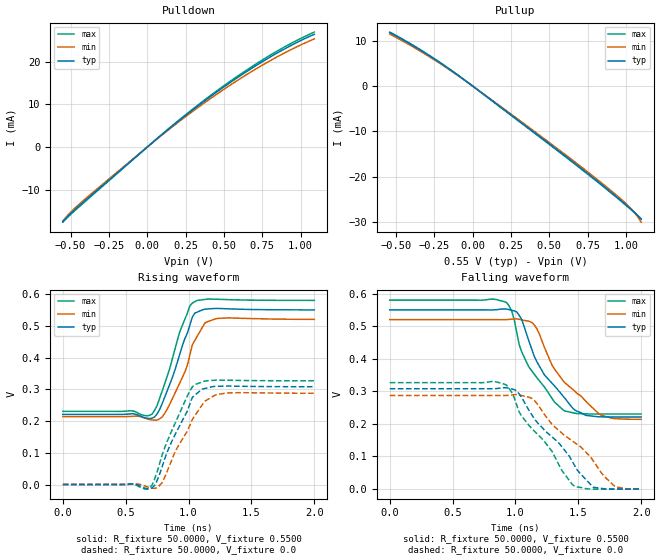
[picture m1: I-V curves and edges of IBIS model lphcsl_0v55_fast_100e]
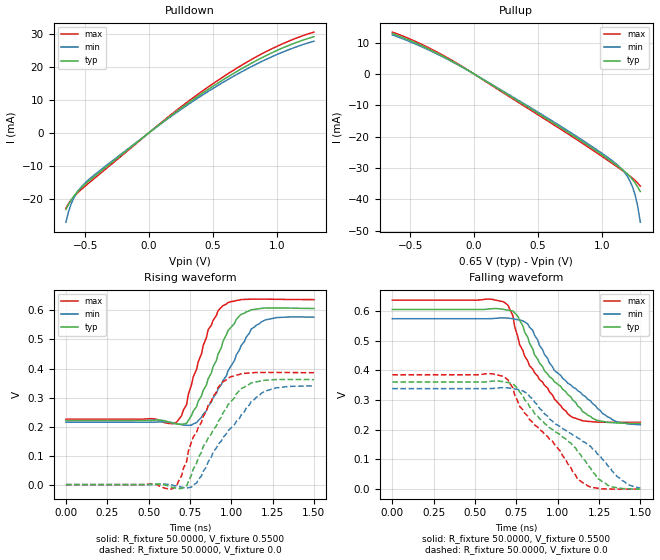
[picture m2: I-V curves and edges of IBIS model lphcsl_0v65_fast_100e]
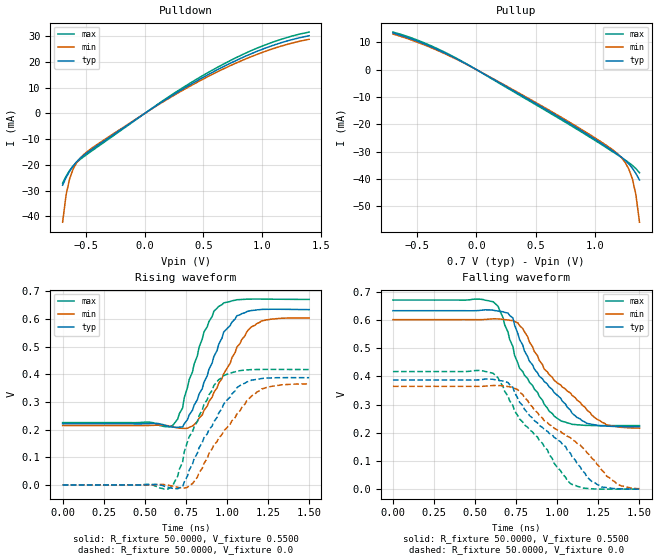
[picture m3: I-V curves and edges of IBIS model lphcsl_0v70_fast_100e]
| Integrated Devices Technolgy, Inc
[IBIS Ver]   4.1
[File name]   9fgl08p1.ibs
[File Rev]   1.0
|Rev history   1.0   original ibis data
[Date]   17 March, 2016
[Disclaimer] Integrated Device Technology, Inc. ("IDT") hereby grants the
   user of this ibis model a non-exclusive, nontransferable
   license to use this ibis model under the following terms. the
   user is granted this license only to use the ibis model and is
   not granted rights to sell, copy (except as needed to run the
   ibis model), rent, lease or sub-license the ibis model in
   whole or in part, or in modified form to anyone. the user may
   modify the ibis model to suit its specific applications, but
   rights to derivative works and such modifications shall belong
   to idt. this ibis model is provided on an as is" basis and idt
   makes absolutely no warranty with respect to the information
   contained herein. idt disclaims and customer waives all
   warranties, express and implied, including warranties of
   merchantability and fitness for a particular purpose. the
   entire risk as to quality and performance is with the user
   accordingly, in no event shall idt be liable for any direct or
   indirect damages, whether in contract or tort, including any
   lost profits or other incidental, consequential, exemplary, or
   punitive damages arising out of the use or application of the
   ibis model. further, idt reserves the right to make changes
   without notice to any product herein to improve reliability,
   function, or design. idt does not convey any license under
   patent rights or any other intellectual property rights,
   including those of third parties. idt is not obligated to
   provide maintenance or support for the licensed ibis model.
[Copyright]   Copyright 2012, Integrated Devices Technolgy, Inc. all rights
   reserved
[Component]   9fgl08p1
[Manufacturer] Integrated Device Technology, Inc.
[Package]
R_pkg   72.4655m   58.886m   86.045m
L_pkg   1.47175nH   1.11650nH   1.77850nH
C_pkg   0.07747pF   0.07444pF   0.08050pF
[Pin] signal_name  model_name
1   vSS_EN_tri   GND
2   GNDXTAL   GND
3   XIN/CLKIN_25   X1
4   X2   X2
5   VDDXTAL3.3   POWER
6   VDDREF3.3   POWER
7   vSADR/REF3.3   REF
8   GNDREF   GND
9   GNDDIG   GND
10   SCLK_3.3   SCIN
11   SDATA_3.3   SCIN
12   VDDDIG3.3   POWER
13   VDDIO   POWER
14   vOE0#   IN
15   DIF0   LP_HCSL
16   DIF0#   LP_HCSL
17   vOE1#   IN
18   DIF1   LP_HCSL
19   DIF1#   LP_HCSL
20   VDD3.3   POWER
21   VDDIO   POWER
22   GND   GND
23   DIF2   LP_HCSL
24   DIF2#   LP_HCSL
25   vOE2#   IN
26   DIF3   LP_HCSL
27   DIF3#   LP_HCSL
28   vOE3#   IN
29   GNDA   GND
30   VDDA3.3   POWER
31   VDDIO   POWER
32   DIF4   LP_HCSL
33   DIF4#   LP_HCSL
34   vOE4#   IN
35   DIF5   LP_HCSL
36   DIF5#   LP_HCSL
37   vOE5#   IN
38   VDD3.3   POWER
39   VDDIO   POWER
40   GND   GND
41   DIF6   LP_HCSL
42   DIF6#   LP_HCSL
43   vOE6#   IN
44   DIF7   LP_HCSL
45   DIF7#   LP_HCSL
46   vOE7#   IN
47   VDDIO   POWER
48   ^CKPWRGD_PD#   PD
49   ePAD   GND
[Diff Pin]  inv_pin  vdiff tdelay_typ tdelay_min  tdelay_max
15   16   NA   0   0   0
18   19   NA   0   0   0
23   24   NA   0   0   0
26   27   NA   0   0   0
32   33   NA   0   0   0
35   36   NA   0   0   0
41   42   NA   0   0   0
44   45   NA   0   0   0
[Model Selector] LP_HCSL
lphcsl_0v55_fast_33e amplitude 0.55V, slew rate fast, 33 ohm diff impedance
lphcsl_0v55_slow_33e amplitude 0.55V, slew rate slow, 33 ohm diff impedance
lphcsl_0v65_fast_33e amplitude 0.65V, slew rate fast, 33 ohm diff impedance
lphcsl_0v65_slow_33e amplitude 0.65V, slew rate slow, 33 ohm diff impedance
lphcsl_0v70_fast_33e amplitude 0.70V, slew rate fast, 33 ohm diff impedance
lphcsl_0v70_slow_33e amplitude 0.70V, slew rate slow, 33 ohm diff impedance
lphcsl_0v80_fast_33e amplitude 0.80V, slew rate fast, 33 ohm diff impedance
lphcsl_0v80_slow_33e amplitude 0.80V, slew rate slow, 33 ohm diff impedance
lphcsl_0v55_fast_85e amplitude 0.55V, slew rate fast, 85 ohm diff impedance
lphcsl_0v55_slow_85e amplitude 0.55V, slew rate slow, 85 ohm diff impedance
lphcsl_0v65_fast_85e amplitude 0.65V, slew rate fast, 85 ohm diff impedance
lphcsl_0v65_slow_85e amplitude 0.65V, slew rate slow, 85 ohm diff impedance
lphcsl_0v70_fast_85e amplitude 0.70V, slew rate fast, 85 ohm diff impedance
lphcsl_0v70_slow_85e amplitude 0.70V, slew rate slow, 85 ohm diff impedance
lphcsl_0v80_fast_85e amplitude 0.80V, slew rate fast, 85 ohm diff impedance
lphcsl_0v80_slow_85e amplitude 0.80V, slew rate slow, 85 ohm diff impedance
lphcsl_0v55_fast_100e amplitude 0.55V, slew rate fast, 100 ohm diff impedance
lphcsl_0v55_slow_100e amplitude 0.55V, slew rate slow, 100 ohm diff impedance
lphcsl_0v65_fast_100e amplitude 0.65V, slew rate fast, 100 ohm diff impedance
lphcsl_0v65_slow_100e amplitude 0.65V, slew rate slow, 100 ohm diff impedance
lphcsl_0v70_fast_100e amplitude 0.70V, slew rate fast, 100 ohm diff impedance
lphcsl_0v70_slow_100e amplitude 0.70V, slew rate slow, 100 ohm diff impedance
lphcsl_0v80_fast_100e amplitude 0.80V, slew rate fast, 100 ohm diff impedance
lphcsl_0v80_slow_100e amplitude 0.80V, slew rate slow, 100 ohm diff impedance
| Models and submodels in the file (30): REF (Output), lphcsl_0v55_fast_100e (Output), lphcsl_0v55_slow_100e (Output), lphcsl_0v65_fast_100e (Output), lphcsl_0v65_slow_100e (Output), lphcsl_0v70_fast_100e (Output), lphcsl_0v70_slow_100e (Output), lphcsl_0v80_fast_100e (Output), lphcsl_0v80_slow_100e (Output), lphcsl_0v55_fast_85e (Output), lphcsl_0v55_slow_85e (Output), lphcsl_0v65_fast_85e (Output), lphcsl_0v65_slow_85e (Output), lphcsl_0v70_fast_85e (Output), lphcsl_0v70_slow_85e (Output), lphcsl_0v80_fast_85e (Output), lphcsl_0v80_slow_85e (Output), lphcsl_0v55_fast_33e (Output), lphcsl_0v55_slow_33e (Output), lphcsl_0v65_fast_33e (Output), lphcsl_0v65_slow_33e (Output), lphcsl_0v70_fast_33e (Output), lphcsl_0v70_slow_33e (Output), lphcsl_0v80_fast_33e (Output), lphcsl_0v80_slow_33e (Output), SCIN (Input), IN (Input), PD (Input), X1 (Input), X2 (Output)
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[Model]   lphcsl_0v55_fast_100e
Model_type Output
Polarity   Non-Inverting
Enable   Active-High
Vmeas =  0.4000V
Cref =   2.0000pF
Rref =   0.0
Vref =   0.4000V
C_comp   1.1000pF   1.0000pF   1.2000pF
[Temperature Range]   25.0000   85.0000   -40.0
[Voltage Range]   0.5500V   0.5200V   0.5800V
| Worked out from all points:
|   slope of the pulldown table from 0 to 0.083 V, typ, clamps not added: 32.7 ohm
|   slope of the pullup table from 0 to 0.083 V, typ, clamps not added: 39.3 ohm
|   rising waveform, R_fixture 50.0000, V_fixture 0.5500: 20-80 % time 174ps typ, 180ps min, 165ps max; typ from 0.221 V to 0.55 V
|   rising waveform, R_fixture 50.0000, V_fixture 0.0: 20-80 % time 210ps typ, 226ps min, 201ps max; typ from 0 V to 0.308 V
|   falling waveform, R_fixture 50.0000, V_fixture 0.5500: 20-80 % time 295ps typ, 339ps min, 258ps max; typ from 0.55 V to 0.221 V
|   falling waveform, R_fixture 50.0000, V_fixture 0.0: 20-80 % time 385ps typ, 441ps min, 351ps max; typ from 0.308 V to 0 V
[Pulldown]
|Voltage   I(typ)   I(min)   I(max)
-550mV    -17.42mA   -17.31mA   -17.56mA
-510mV    -15.92mA   -15.61mA   -16.12mA
-470mV    -14.59mA   -14.21mA   -14.8mA
-310mV    -9.584mA   -9.264mA   -9.753mA
90mV      2.747mA    2.637mA    2.806mA
350mV     10.16mA    9.756mA    10.37mA
570mV     15.8mA     15.17mA    16.12mA
750mV     19.95mA    19.15mA    20.36mA
910mV     23.24mA    22.29mA    23.72mA
1.09V     26.39mA    25.32mA    26.91mA
[Pullup]
|Voltage   I(typ)   I(min)   I(max)
-540mV    11.78mA    11.45mA    11.88mA
-360mV    8.313mA    8.057mA    8.417mA
-160mV    3.912mA    3.778mA    3.974mA
0V        -107.6pA   -683pA     -85.53pA
480mV     -12.23mA   -11.94mA   -12.36mA
760mV     -19.55mA   -19.19mA   -19.69mA
960mV     -25.05mA   -24.7mA    -25.17mA
1.04V     -27.39mA   -27.28mA   -27.47mA
1.08V     -28.69mA   -28.98mA   -28.66mA
1.1V      -29.42mA   -30.05mA   -29.29mA
[Ramp]
| variable   typ   min   max
dV/dt_r  0.1848/0.2165n   0.1724/0.2461n   0.1960/0.2011n
dV/dt_f  0.1973/0.2848n   0.1835/0.3291n   0.2098/0.2758n
R_load = 50.0000
[Rising Waveform]
R_fixture= 50.0000
V_fixture= 0.5500
V_fixture_min= 0.5200
V_fixture_max= 0.5800
|time   V(typ)   V(min)   V(max)
0s        221mV      213.9mV    230.4mV
710ps     208.9mV    203.3mV    222mV
770ps     236.5mV    207.1mV    271.8mV
830ps     295.1mV    237.4mV    341.4mV
930ps     410.6mV    320mV      481.3mV
1.01ns    502mV      407.6mV    562.8mV
1.07ns    543.3mV    467.9mV    580.1mV
1.13ns    552.4mV    509.1mV    583mV
1.23ns    554.6mV    523.3mV    583.5mV
2ns       550.1mV    520.2mV    580mV
[Rising Waveform]
R_fixture= 50.0000
V_fixture= 0.0
V_fixture_min= 0.0
V_fixture_max= 0.0
|time   V(typ)   V(min)   V(max)
0s        0V         0V         0V
690ps     -13.76mV   -9.908mV   -11mV
730ps     -2.555mV   -12mV      17.28mV
790ps     56.31mV    6.206mV    93.42mV
890ps     155mV      100.6mV    190.4mV
990ps     231mV      167.8mV    278.9mV
1.05ns    281.3mV    216.8mV    314.6mV
1.13ns    302.4mV    262.5mV    326.1mV
1.23ns    309.3mV    283.7mV    328.7mV
2ns       308mV      287.4mV    326.7mV
[Falling Waveform]
R_fixture= 50.0000
V_fixture= 0.5500
V_fixture_min= 0.5200
V_fixture_max= 0.5800
|time   V(typ)   V(min)   V(max)
0s        550mV      520mV      580mV
930ps     552.4mV    520.1mV    572.5mV
970ps     548.8mV    521.6mV    546.6mV
1.03ns    533mV      521mV      442.9mV
1.11ns    451.2mV    514.7mV    373mV
1.23ns    350.6mV    435.4mV    313.4mV
1.31ns    317mV      368.9mV    267.2mV
1.47ns    243.2mV    301.1mV    233mV
1.68ns    221.7mV    226.8mV    230.4mV
2ns       221.1mV    214.1mV    230.4mV
[Falling Waveform]
R_fixture= 50.0000
V_fixture= 0.0
V_fixture_min= 0.0
V_fixture_max= 0.0
|time   V(typ)   V(min)   V(max)
0s        307.9mV    287.3mV    326.7mV
890ps     310.7mV    287.1mV    324.6mV
950ps     309.3mV    287.8mV    308.9mV
1.01ns    301.5mV    290mV      257.9mV
1.11ns    240.4mV    281.8mV    194.3mV
1.29ns    160.4mV    199.1mV    116.1mV
1.47ns    72.59mV    142.7mV    8.438mV
1.62ns    5.493mV    86.02mV    77.42uV
1.78ns    -65.96uV   11.35mV    -85.75uV
2ns       -77.45uV   -198.5uV   -34.61uV
[Model]   lphcsl_0v65_fast_100e
Model_type Output
Polarity   Non-Inverting
Enable   Active-High
Vmeas =  0.4000V
Cref =   2.0000pF
Rref =   0.0
Vref =   0.4000V
C_comp   1.1000pF   1.0000pF   1.2000pF
[Temperature Range]   25.0000   85.0000   -40.0000
[Voltage Range]   0.6500V   0.6200V   0.6800V
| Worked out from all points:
|   slope of the pulldown table from 0 to 0.098 V, typ, clamps not added: 32.8 ohm
|   slope of the pullup table from 0 to 0.098 V, typ, clamps not added: 40 ohm
|   rising waveform, R_fixture 50.0000, V_fixture 0.5500: 20-80 % time 168ps typ, 206ps min, 144ps max; typ from 0.221 V to 0.607 V
|   rising waveform, R_fixture 50.0000, V_fixture 0.0: 20-80 % time 214ps typ, 251ps min, 168ps max; typ from 0 V to 0.362 V
|   falling waveform, R_fixture 50.0000, V_fixture 0.5500: 20-80 % time 294ps typ, 332ps min, 239ps max; typ from 0.606 V to 0.222 V
|   falling waveform, R_fixture 50.0000, V_fixture 0.0: 20-80 % time 376ps typ, 429ps min, 326ps max; typ from 0.361 V to 0 V
[Pulldown]
|Voltage   I(typ)   I(min)   I(max)
-650mV    -23.23mA   -27.08mA   -22.85mA
-630mV    -21.73mA   -23.92mA   -21.53mA
-610mV    -20.42mA   -21.63mA   -20.41mA
-590mV    -19.28mA   -19.88mA   -19.45mA
-550mV    -17.42mA   -17.37mA   -17.87mA
-510mV    -15.92mA   -15.58mA   -16.5mA
-350mV    -10.82mA   -10.4mA    -11.34mA
130mV     3.938mA    3.75mA     4.173mA
450mV     12.8mA     12.19mA    13.51mA
770mV     20.38mA    19.39mA    21.48mA
1.03V     25.42mA    24.16mA    26.67mA
1.29V     29.08mA    27.71mA    30.47mA
[Pullup]
|Voltage   I(typ)   I(min)   I(max)
-640mV    12.9mA     12.48mA    13.37mA
-340mV    7.668mA    7.369mA    8.057mA
-40mV     988uA      943.5uA    1.052mA
700mV     -17.66mA   -17.23mA   -18.19mA
1.08V     -28.05mA   -27.62mA   -28.49mA
1.16V     -30.49mA   -30.54mA   -30.78mA
1.2V      -31.91mA   -32.71mA   -31.96mA
1.22V     -32.74mA   -34.19mA   -32.58mA
1.24V     -33.69mA   -36.08mA   -33.24mA
1.26V     -34.78mA   -38.62mA   -33.96mA
1.28V     -36.03mA   -42.17mA   -34.78mA
1.3V      -37.46mA   -47.25mA   -35.74mA
[Ramp]
| variable   typ   min   max
dV/dt_r  0.2171/0.2129n   0.2039/0.2456n   0.2314/0.1862n
dV/dt_f  0.2322/0.2706n   0.2162/0.3099n   0.2487/0.2338n
R_load = 50.0000
[Rising Waveform]
R_fixture= 50.0000
V_fixture= 0.5500
V_fixture_min= 0.5200
V_fixture_max= 0.5800
|time   V(typ)   V(min)   V(max)
0s        221mV      214.9mV    225.3mV
650ps     210.5mV    212.1mV    210.1mV
730ps     211.4mV    204.5mV    276.1mV
790ps     268.6mV    213.4mV    396.8mV
860ps     364.5mV    269.7mV    533.4mV
950ps     494mV      359.2mV    616.5mV
1.05ns    581.6mV    464.5mV    635.9mV
1.15ns    604.7mV    548.6mV    639.1mV
1.27ns    608.6mV    575.2mV    638.3mV
1.5ns     606.8mV    576.9mV    637.3mV
[Rising Waveform]
R_fixture= 50.0000
V_fixture= 0.0
V_fixture_min= 0.0
V_fixture_max= 0.0
|time   V(typ)   V(min)   V(max)
0s        0V         0V         0V
640ps     -8.434mV   -704uV     -15.02mV
700ps     -13.35mV   -8.846mV   31.11mV
730ps     -5.209mV   -11.48mV   79.09mV
760ps     34.44mV    -8.318mV   147.9mV
790ps     73.04mV    5.508mV    180.3mV
950ps     247.4mV    162.6mV    354.6mV
1.06ns    330.8mV    239.9mV    381.8mV
1.2ns     359.3mV    320.7mV    386.4mV
1.5ns     361.8mV    339.9mV    385.6mV
[Falling Waveform]
R_fixture= 50.0000
V_fixture= 0.5500
V_fixture_min= 0.5200
V_fixture_max= 0.5800
|time   V(typ)   V(min)   V(max)
0s        605.5mV    574.4mV    637mV
610ps     608.4mV    574.9mV    639.2mV
730ps     600.1mV    574.5mV    584.1mV
770ps     569.5mV    570.1mV    487.1mV
830ps     491.6mV    545.6mV    416.2mV
920ps     399.1mV    454.6mV    350.4mV
1.06ns    319.5mV    357.6mV    254.3mV
1.23ns    233.7mV    280.6mV    226.2mV
1.36ns    223mV      226.1mV    225.3mV
1.5ns     221.5mV    216.9mV    225.3mV
[Falling Waveform]
R_fixture= 50.0000
V_fixture= 0.0
V_fixture_min= 0.0
V_fixture_max= 0.0
|time   V(typ)   V(min)   V(max)
0s        361mV      338.8mV    385.4mV
610ps     364mV      339.3mV    388.2mV
680ps     360.8mV    341.6mV    377mV
730ps     355.5mV    339.4mV    341.2mV
770ps     327.7mV    334.4mV    279.2mV
970ps     200.9mV    228.4mV    160.8mV
1.12ns    126.5mV    172.8mV    33.06mV
1.3ns     13.89mV    80.88mV    422.7uV
1.42ns    1.232mV    16.25mV    -179.8uV
1.5ns     169.3uV    3.586mV    -100uV
[Model]   lphcsl_0v70_fast_100e
Model_type Output
Polarity   Non-Inverting
Enable   Active-High
Vmeas =  0.4000V
Cref =   2.0000pF
Rref =   0.0
Vref =   0.4000V
C_comp   1.1000pF   1.0000pF   1.2000pF
[Temperature Range]   25.0000   85.0000   -40.0000
[Voltage Range]   0.7000V   0.6700V   0.7400V
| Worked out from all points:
|   slope of the pulldown table from 0 to 0.105 V, typ, clamps not added: 32.9 ohm
|   slope of the pullup table from 0 to 0.105 V, typ, clamps not added: 40.5 ohm
|   rising waveform, R_fixture 50.0000, V_fixture 0.5500: 20-80 % time 164ps typ, 205ps min, 146ps max; typ from 0.221 V to 0.634 V
|   rising waveform, R_fixture 50.0000, V_fixture 0.0: 20-80 % time 214ps typ, 252ps min, 170ps max; typ from 0 V to 0.388 V
|   falling waveform, R_fixture 50.0000, V_fixture 0.5500: 20-80 % time 286ps typ, 333ps min, 230ps max; typ from 0.633 V to 0.221 V
|   falling waveform, R_fixture 50.0000, V_fixture 0.0: 20-80 % time 372ps typ, 416ps min, 296ps max; typ from 0.387 V to 0 V
[Pulldown]
|Voltage   I(typ)   I(min)   I(max)
-700mV    -27.91mA   -42.29mA   -27.13mA
-670mV    -24.93mA   -31.58mA   -24.4mA
-640mV    -22.46mA   -25.38mA   -22.16mA
-610mV    -20.43mA   -21.63mA   -20.41mA
-550mV    -17.42mA   -17.37mA   -17.87mA
-460mV    -14.27mA   -13.81mA   -14.87mA
170mV     5.111mA    4.867mA    5.413mA
620mV     17mA       16.18mA    17.92mA
830mV     21.65mA    20.59mA    22.8mA
1.01V     25.07mA    23.84mA    26.32mA
1.22V     28.24mA    26.89mA    29.6mA
1.4V      30.17mA    28.8mA     31.59mA
[Pullup]
|Voltage   I(typ)   I(min)   I(max)
-700mV    13.37mA    12.97mA    13.69mA
-400mV    8.685mA    8.356mA    9.067mA
-40mV     976.3uA    932.1uA    1.037mA
710mV     -17.77mA   -17.34mA   -18.25mA
1.01V     -25.83mA   -25.34mA   -26.25mA
1.16V     -30.15mA   -29.81mA   -30.44mA
1.22V     -32.05mA   -32.24mA   -32.17mA
1.25V     -33.15mA   -33.95mA   -33.06mA
1.28V     -34.44mA   -36.32mA   -33.98mA
1.31V     -36.02mA   -39.87mA   -35mA
1.34V     -37.97mA   -45.72mA   -36.19mA
1.37V     -40.34mA   -55.75mA   -37.7mA
[Ramp]
| variable   typ   min   max
dV/dt_r  0.2327/0.2120n   0.2192/0.2438n   0.2503/0.1864n
dV/dt_f  0.2497/0.2565n   0.2337/0.2967n   0.2701/0.2197n
R_load = 50.0000
[Rising Waveform]
R_fixture= 50.0000
V_fixture= 0.5500
V_fixture_min= 0.5200
V_fixture_max= 0.5800
|time   V(typ)   V(min)   V(max)
0s        221mV      214.9mV    225.3mV
650ps     210.9mV    212.4mV    210.2mV
730ps     209.9mV    204.6mV    278mV
800ps     288.3mV    217.9mV    436.5mV
860ps     371.3mV    269.2mV    553.3mV
950ps     508.9mV    368mV      645.7mV
1.06ns    611.8mV    498mV      669.8mV
1.15ns    630.9mV    572mV      672.2mV
1.24ns    635.1mV    597mV      672mV
1.5ns     634mV      603.5mV    671mV
[Rising Waveform]
R_fixture= 50.0000
V_fixture= 0.0
V_fixture_min= 0.0
V_fixture_max= 0.0
|time   V(typ)   V(min)   V(max)
0s        0V         0V         0V
640ps     -8.091mV   -315uV     -15.03mV
670ps     -12.45mV   -4.428mV   -2.669mV
730ps     -7.069mV   -11.24mV   81.56mV
770ps     53.48mV    -3.061mV   174.1mV
860ps     170.1mV    77.73mV    291.3mV
980ps     292.4mV    195mV      395.2mV
1.09ns    363.9mV    280.3mV    414.1mV
1.21ns    384.8mV    347.2mV    417.7mV
1.5ns     387.8mV    365.3mV    417.2mV
[Falling Waveform]
R_fixture= 50.0000
V_fixture= 0.5500
V_fixture_min= 0.5200
V_fixture_max= 0.5800
|time   V(typ)   V(min)   V(max)
0s        632.9mV    601.2mV    670.7mV
610ps     634.7mV    604mV      664.5mV
640ps     631.8mV    603.8mV    648.2mV
730ps     606.8mV    597.8mV    505.4mV
770ps     531.2mV    580.1mV    429.2mV
830ps     454.4mV    522.4mV    379.2mV
950ps     363mV      406.2mV    276.6mV
1.12ns    254.1mV    315.7mV    228.3mV
1.3ns     223.5mV    227.5mV    225.4mV
1.5ns     221.4mV    216.3mV    225.3mV
[Falling Waveform]
R_fixture= 50.0000
V_fixture= 0.0
V_fixture_min= 0.0
V_fixture_max= 0.0
|time   V(typ)   V(min)   V(max)
0s        387.1mV    364.6mV    417.1mV
610ps     389.4mV    367.5mV    410.7mV
730ps     361.1mV    361.3mV    296.8mV
830ps     261mV      302.3mV    210.9mV
920ps     212mV      242.7mV    151.3mV
1.08ns    127mV      182.3mV    19.84mV
1.18ns    43.36mV    129.4mV    2.496mV
1.27ns    7.62mV     67.37mV    132.2uV
1.38ns    1.242mV    13.5mV     -120.3uV
1.5ns     113.4uV    1.53mV     -45.16uV
